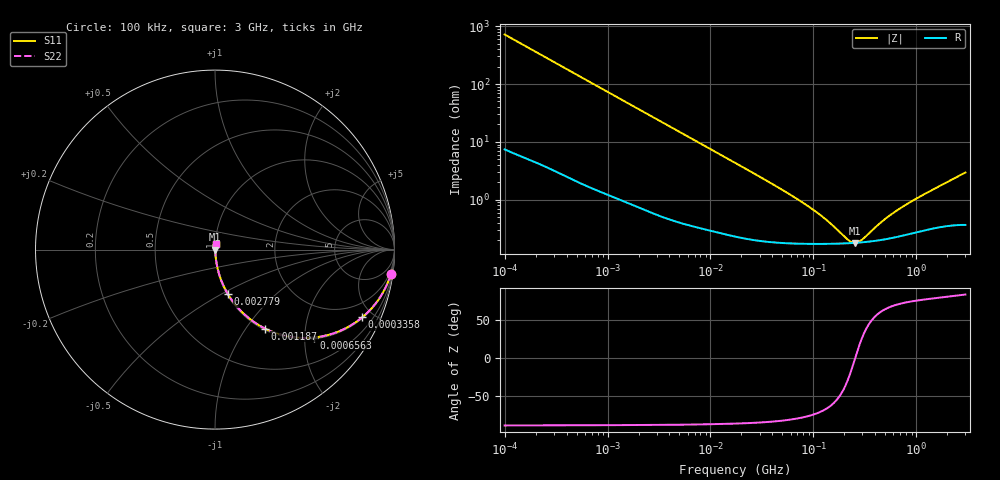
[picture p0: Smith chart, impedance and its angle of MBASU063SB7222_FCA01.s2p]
! MBASU063SB7222_FCA01  S-PARAMETER MODEL  ( Standard Model )
! Model Generated by TAIYO YUDEN Corporation (https://www.yuden.co.jp/en/)
! Version 1.0
! TAIYO YUDEN Control No. 250312
! Copyright(c) 2025 TAIYO YUDEN CO.,LTD. All Rights Reserved.
! Product Description (link to TY-COMPAS)
! https://ds.yuden.co.jp/TYCOMPAS/or/detail?pn=MBASU063SB7222KFCA01&u=M
! Products Name : Multilayer Ceramic Capacitors
! Characteristics :
!  Capacitance : 2200 [pF] , Rated Voltage : 50 [V] , TCC : X7R
!  Case Size : 0.6 x 0.3 / 0.024 x 0.012 [mm/inch] , Thickness : 0.3 / 0.012 [mm/inch]
!  (Conditions: Temperature = 25 [degC] , DC Bias Voltage = 0 [V])
! External Node Assignments :
!  1  o---| |---o  2
! GND o---------o GND
! Frequency Range : 100kHz  -  3GHz  [ 401 STEP ]
# MHZ S RI R 50
! Freq[MHz].  S11 Real  S11 Imag  S21 Real  S21 Imag  S12 Real  S12 Imag  S22 Real  S22 Imag
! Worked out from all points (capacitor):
!   401 points, 100 kHz to 3 GHz, reference 50 ohm
!   read as one part in series: C = 2.21 nF near 105.3 kHz
!   lowest |Z| = 179 mohm at 252.7 MHz (marker M1)
!   series resonance near 255.8 MHz, so ESL is about 180 pH
!   S11 on the Smith chart (normalised r, x): 100 kHz: 1, -14; 335.8 kHz: 1.06, -4.32; 656.3 kHz: 1.03, -2.22; 1.187 MHz: 1.02, -1.24; 2.779 MHz: 1.01, -0.53; 3 GHz: 1.01, +0.06
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0.1  0.9797 -0.1359  0.0203 0.1359  0.0203 0.1359  0.9797 -0.1359
0.200542  0.9259 -0.2559  0.0741 0.2559  0.0741 0.2559  0.9259 -0.2559
0.335785  0.8205 -0.3771  0.1795 0.3771  0.1795 0.3771  0.8205 -0.3771
0.562235  0.6253 -0.4769  0.3747 0.4769  0.3747 0.4769  0.6253 -0.4769
0.656258  0.5523 -0.4899  0.4477 0.4899  0.4477 0.4899  0.5523 -0.4899
0.871356  0.4149 -0.4848  0.5851 0.4848  0.5851 0.4848  0.4149 -0.4848
1.18716  0.2799 -0.4403  0.7201 0.4403  0.7201 0.4403  0.2799 -0.4403
1.793056  0.1494 -0.3469  0.8506 0.3469  0.8506 0.3469  0.1494 -0.3469
2.778892  0.0709 -0.2461  0.9291 0.2461  0.9291 0.2461  0.0709 -0.2461
3.161081  0.0566 -0.2201  0.9434 0.2201  0.9434 0.2201  0.0566 -0.2201
6.848882  0.015 -0.107  0.985 0.107  0.985 0.107  0.015 -0.107
17.7727  0.00405 -0.0421  0.9959 0.0421  0.9959 0.0421  0.00405 -0.0421
51.12795  0.00198 -0.0142  0.998 0.0142  0.998 0.0142  0.00198 -0.0142
97.38194  0.00176 -0.00667  0.9982 0.00667  0.9982 0.00667  0.00176 -0.00667
139.694  0.00173 -0.00381  0.9983 0.00381  0.9983 0.00381  0.00173 -0.00381
216.4987  0.00176 -0.000989  0.9982 0.000989  0.9982 0.000989  0.00176 -0.000989
252.704  0.00179 -7.11e-05  0.9982 7.11e-05  0.9982 7.11e-05  0.00179 -7.11e-05
294.964  0.00183 0.000841  0.9982 -0.000841  0.9982 -0.000841  0.00183 0.000841
434.1712  0.00199 0.00322  0.998 -0.00322  0.998 -0.00322  0.00199 0.00322
547.5153  0.00215 0.00481  0.9979 -0.00481  0.9979 -0.00481  0.00215 0.00481
1016.304  0.00284 0.0102  0.9972 -0.0102  0.9972 -0.0102  0.00284 0.0102
3000  0.00449 0.0291  0.9955 -0.0291  0.9955 -0.0291  0.00449 0.0291
